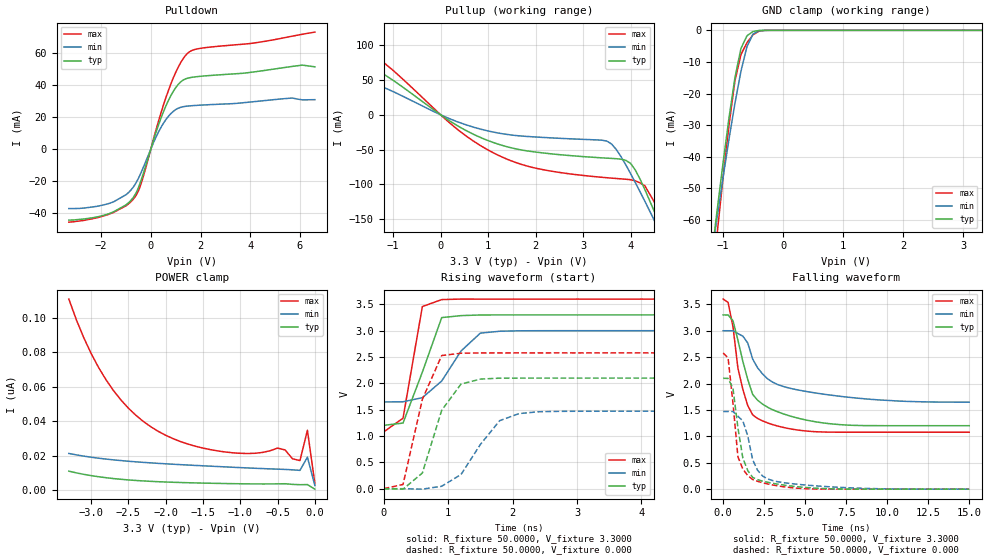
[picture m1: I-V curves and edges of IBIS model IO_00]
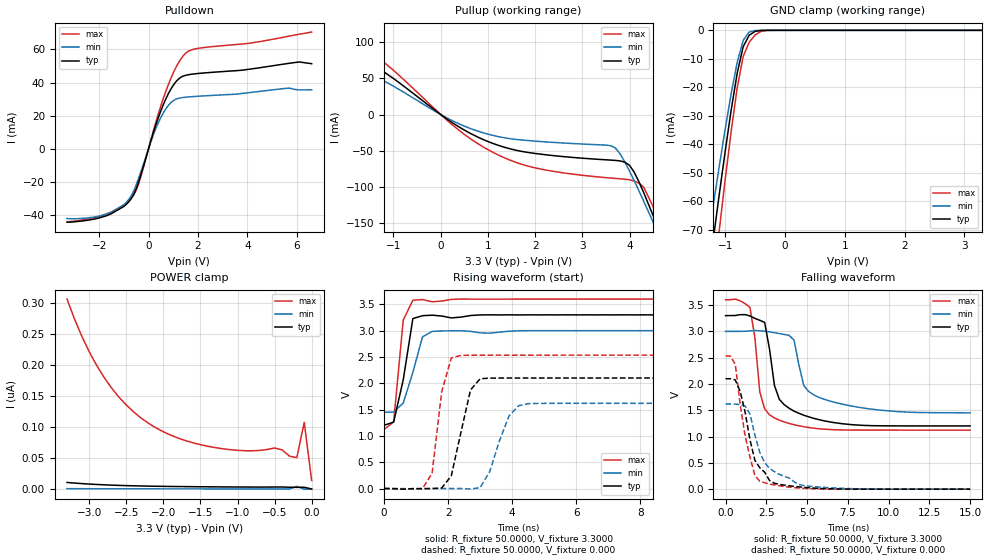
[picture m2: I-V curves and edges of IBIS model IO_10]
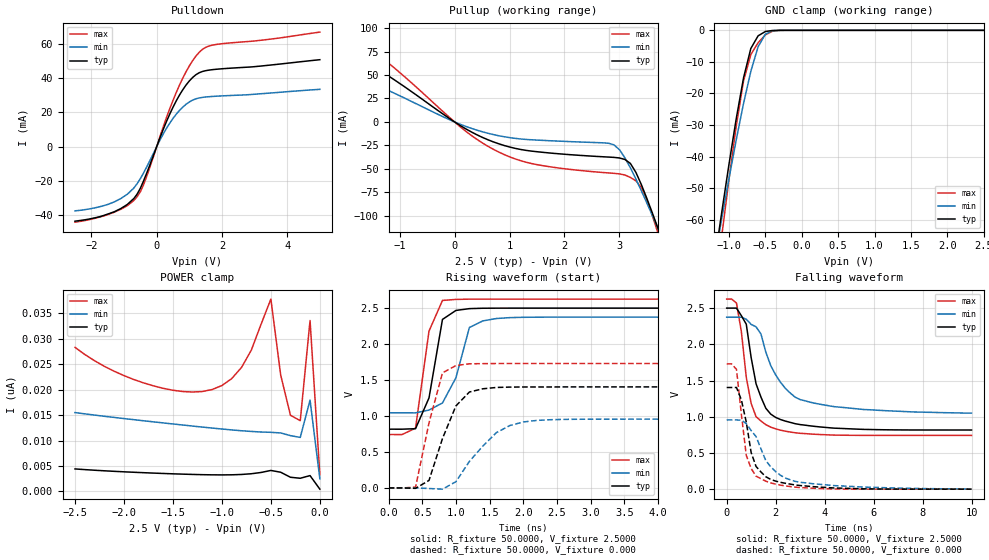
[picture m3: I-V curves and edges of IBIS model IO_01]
| Xilinx XC9500XV IBIS File
[IBIS ver]   2.1
[File name]   xc9500xv.ibs
[File Rev]   0.2
[Date]   Mar. 6, 2001
[Source]   Hspice simulations
[Notes]   Xilinx IBIS model for XC9500XV I/O
|   The package models are provided for CS48, PC44, VQ44
|   TQ100, TQ144, CS144, PQ208, FG256, and CS280 package
|   types, with CS48 being selected as a default. Please
|   make your own selection of the packages by commenting
|   out the unused ones.
|   Control flag setting:
|   SLW=0 - fast slew rate
|   SLW=1 - slow slew rate
|   VIO=2 - 1.8V Vddio
|   VIO=1 - 2.5V Vddio
|   VIO=0 - 3.3V Vddio
|   COMMENTS: Models include process corners for MIN and MAX.
[Disclaimer]   The data in this model is derived from SPICE simulations
|   using modeling information extracted from the target pro-
|   cess. While a great deal of care has been take to provide
|   information that is accurate, this model is considered
|   preliminary as it has not been verified by actual silicon
|   measurement. Treat the data in this model as preliminary
|   until actual silicon verification is performed.
[Copyright]   Copyright 2001, Xilinx Inc., All rights reserved
|   Component XC9500XV
|   >>> Make Your Selection of the Package type Below <<<
[Component]   XC9500XV
[Manufacturer]   Xilinx Inc.
[Package]
| For package type CS48:
| variable   typ   min   max
R_pkg   112.000m   98.0000m   126.000m
L_pkg   2.1000nH   1.8000nH   2.4000nH
C_pkg   0.2500pF   0.2000pF   0.3000pF
| For package type PC44:
| variable   typ   min   max
|R_pkg   67.5000m   66.0000m   69.0000m
|L_pkg   3.9500nH   3.6000nH   4.3000nH
|C_pkg   0.9000pF   0.8000pF   1.0000pF
| For package type VQ44:
| variable   typ   min   max
|R_pkg   57.0000m   54.0000m   60.0000m
|L_pkg   2.2500nH   2.1000nH   2.4000nH
|C_pkg   0.3000pF   0.3000pF   0.3000pF
| For package type TQ100:
| variable   typ   min   max
|R_pkg   103.000m   98.0000m   108.000m
|L_pkg   5.3000nH   4.7000nH   5.9000nH
|C_pkg   0.5500pF   0.4000pF   0.7000pF
| For package type TQ144:
| variable   typ   min   max
|R_pkg   127.000m   117.000m   137.000m
|L_pkg   8.1500nH   7.1000nH   9.2000nH
|C_pkg   1.0500pF   0.8000pF   1.3000pF
| For package type CS144:
| variable   typ   min   max
|R_pkg   109.500m   76.0000m   143.000m
|L_pkg   2.2500nH   1.5000nH   3.0000nH
|C_pkg   0.2500pF   0.2000pF   0.3000pF
| For package type PQ208:
| variable   typ   min   max
|R_pkg   195.500m   195.000m   196.000m
|L_pkg   14.200nH   12.500nH   15.900nH
|C_pkg   1.8000pF   1.6000pF   2.0000pF
| For package type FG256:
| variable   typ   min   max
|R_pkg   185.500m   141.000m   230.000m
|L_pkg   4.8500nH   3.3000nH   6.4000nH
|C_pkg   0.7500pF   0.5000pF   1.0000pF
| For package type CS280:
| variable   typ   min   max
|R_pkg   259.500m   148.000m   371.000m
|L_pkg   5.8000nH   2.7000nH   8.9000nH
|C_pkg   0.5000pF   0.2000pF   0.8000pF
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[Pin]  signal_name   model_name   R_pin   L_pin   C_pin
io_0   io_0   IO_00   NA   NA   NA
io_1   io_1   IO_01   NA   NA   NA
io_2   io_2   IO_10   NA   NA   NA
io_3   io_3   IO_11   NA   NA   NA
io_4   io_4   IO_02   NA   NA   NA
io_5   io_5   IO_12   NA   NA   NA
VCCO   VCCO   POWER   NA   NA   NA
PGND   GND   GND   NA   NA   NA
| Models and submodels in the file (6): IO_00 (I/O), IO_10 (I/O), IO_01 (I/O), IO_11 (I/O), IO_02 (I/O), IO_12 (I/O)
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|   Model IO_00
[Model]   IO_00
Model_type   I/O
Polarity   Non-Inverting
Enable   Active-High
Vinl =   0.8000V
Vinh =   2.0000V
Vmeas =   1.5000V
Cref =  50.0000pF
Rref =   1.0000M
Vref =  0.000V
C_comp   1.8820pF   1.2910pF   2.4730pF
[Temperature Range]   25.0000   100.0000   0.000
[Voltage Range]   3.3000V   3.0000V   3.6000V
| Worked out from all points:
|   slope of the pulldown table from 0 to 0.495 V, typ, clamps not added: 21.7 ohm
|   slope of the pullup table from 0 to 0.495 V, typ, clamps not added: 23.3 ohm
|   GND clamp passes 1 mA (typ) near -0.55 V on its own axis
|   rising waveform, R_fixture 50.0000, V_fixture 3.3000: 20-80 % time 377ps typ, 522ps min, 214ps max; typ from 1.2 V to 3.3 V
|   rising waveform, R_fixture 50.0000, V_fixture 0.000: 20-80 % time 385ps typ, 511ps min, 351ps max; typ from 0 V to 2.1 V
|   falling waveform, R_fixture 50.0000, V_fixture 3.3000: 20-80 % time 1.51ns typ, 2.44ns min, 914ps max; typ from 3.3 V to 1.2 V
|   falling waveform, R_fixture 50.0000, V_fixture 0.000: 20-80 % time 721ps typ, 953ps min, 579ps max; typ from 2.1 V to 0 V
[Pulldown]
| voltage   I(typ)   I(min)   I(max)
-3.3V     -44.4mA    -37.2mA    -45.7mA
-1.5V     -39.2mA    -33mA      -39.6mA
-900mV    -33.61mA   -27.22mA   -34.3mA
-600mV    -27.65mA   -21.23mA   -29.11mA
-400mV    -19.86mA   -14.99mA   -22.06mA
200mV     10.04mA    7.201mA    11.53mA
600mV     26.71mA    18.26mA    31.83mA
1.1V      40.32mA    25.49mA    51.09mA
1.5V      44.33mA    26.86mA    60.13mA
2V        45.44mA    27.42mA    62.92mA
6.1V      52.41mA    30.72mA    71.7mA
6.6V      51.35mA    30.83mA    73.05mA
[Pullup]
| voltage   I(typ)   I(min)   I(max)
-3.3V     27.71mA    12.26mA    53.81mA
-2.5V     82.24mA    44.55mA    121.5mA
-2.3V     93.8mA     55.81mA    126.3mA
-1.7V     79.94mA    53.81mA    102.7mA
300mV     -13.55mA   -8.683mA   -18.05mA
1.2V      -42.02mA   -26.09mA   -57.83mA
3.5V      -62.42mA   -37.86mA   -90.63mA
4V        -69.96mA   -84.71mA   -93.48mA
4.3V      -107.6mA   -124.5mA   -102.2mA
4.5V      -139.2mA   -152.1mA   -125.6mA
4.7V      -172.1mA   -180mA     -161.3mA
6.6V      -491mA     -449mA     -534.4mA
[GND_clamp]
| voltage   I(typ)   I(min)   I(max)
-3.3V     -420.2mA   -364.8mA   -490.5mA
-1.2V     -73.41mA   -72.76mA   -83.75mA
-1.1V     -57.66mA   -59.66mA   -65.15mA
-1V       -42.38mA   -46.89mA   -47.13mA
-900mV    -27.9mA    -34.62mA   -30.25mA
-800mV    -15.03mA   -23.13mA   -16mA
-700mV    -5.736mA   -12.97mA   -7.676mA
-600mV    -1.742mA   -5.18mA    -3.915mA
-500mV    -371uA     -1.195mA   -1.433mA
-400mV    -43.14uA   -156.3uA   -255.7uA
-300mV    -2.671uA   -9.839uA   -22.16uA
3.3V      462pA      11.68nA    3.111nA
[POWER_clamp]
| voltage   I(typ)   I(min)   I(max)
-3.3V     10.92nA    21.19nA    110.8nA
-3.1V     9.067nA    19.64nA    88.41nA
-2.8V     7.101nA    17.92nA    63.87nA
-2.6V     6.191nA    17.05nA    52.17nA
-2.3V     5.238nA    16.01nA    39.75nA
-2V       4.618nA    15.18nA    31.72nA
-1.6V     4.086nA    14.24nA    25.36nA
-900mV    3.547nA    12.78nA    21.16nA
-500mV    3.553nA    12.08nA    24.31nA
-200mV    3.052nA    11.37nA    17.04nA
-100mV    3.12nA     19.04nA    34.64nA
0V        462pA      2.582nA    3.744nA
[Ramp]
| variable   typ   min   max
dV/dt_r   1.2600/0.3171n   0.8826/0.5251n   1.5468/0.2348n
dV/dt_f   1.2588/1.4787n   0.8112/2.5016n   1.5132/0.8154n
R_load = 50.0000
[Rising Waveform]
R_fixture = 50.0000
V_fixture = 3.3000
V_fixture_min = 3.0000
V_fixture_max = 3.6000
L_fixture = 0.000H
C_fixture = 0.000F
| time   V(typ)   V(min)   V(max)
0s        1.202V     1.647V     1.078V
300ps     1.246V     1.65V      1.338V
600ps     2.213V     1.728V     3.458V
900ps     3.248V     2.044V     3.59V
1.2ns     3.286V     2.614V     3.6V
1.5ns     3.298V     2.954V     3.599V
1.8ns     3.299V     2.989V     3.599V
2.7ns     3.3V       2.999V     3.599V
15ns      3.299V     3V         3.599V
[Rising Waveform]
R_fixture = 50.0000
V_fixture = 0.000
V_fixture_min = 0.000
V_fixture_max = 0.000
L_fixture = 0.000H
C_fixture = 0.000F
| time   V(typ)   V(min)   V(max)
0s        7.285uV    -1.674uV   37.74uV
300ps     -9.219mV   -254.7uV   79.99mV
600ps     297.3mV    -9.006mV   1.696V
900ps     1.488V     46.1mV     2.528V
1.2ns     1.986V     269.2mV    2.572V
1.5ns     2.081V     838.4mV    2.577V
1.8ns     2.099V     1.292V     2.577V
2.1ns     2.099V     1.425V     2.578V
2.4ns     2.099V     1.46V      2.577V
15ns      2.1V       1.471V     2.578V
[Falling Waveform]
R_fixture = 50.0000
V_fixture = 3.3000
V_fixture_min = 3.0000
V_fixture_max = 3.6000
L_fixture = 0.000H
C_fixture = 0.000F
| time   V(typ)   V(min)   V(max)
0s        3.3V       3V         3.6V
300ps     3.298V     3V         3.536V
600ps     3.189V     2.999V     3.072V
900ps     2.821V     2.946V     2.292V
1.2ns     2.421V     2.898V     1.889V
1.8ns     1.794V     2.462V     1.407V
2.1ns     1.684V     2.299V     1.338V
3ns       1.506V     2.029V     1.224V
5.1ns     1.306V     1.848V     1.1V
15ns      1.202V     1.648V     1.078V
[Falling Waveform]
R_fixture = 50.0000
V_fixture = 0.000
V_fixture_min = 0.000
V_fixture_max = 0.000
L_fixture = 0.000H
C_fixture = 0.000F
| time   V(typ)   V(min)   V(max)
0s        2.1V       1.471V     2.578V
300ps     2.097V     1.471V     2.486V
600ps     1.907V     1.47V      1.623V
900ps     1.162V     1.381V     612.7mV
1.2ns     586.1mV    1.293V     381mV
1.5ns     351.2mV    1.008V     255.1mV
1.8ns     222.8mV    553.8mV    183mV
2.4ns     152.3mV    250.2mV    122.1mV
3.9ns     69.47mV    114.2mV    37.16mV
15ns      -2.014uV   295.5uV    8.128uV
|   Model IO_10
[Model]   IO_10
Model_type   I/O
Polarity   Non-Inverting
Enable   Active-High
Vinl =   0.8000V
Vinh =   2.0000V
Vmeas =   1.6500V
Cref =  50.0000pF
Rref =   1.0000M
Vref =  0.000V
C_comp   1.8820pF   1.2910pF   2.4730pF
[Temperature Range]   25.0000   100.0000   0.000
[Voltage Range]   3.3000V   3.0000V   3.6000V
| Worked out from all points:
|   slope of the pulldown table from 0 to 0.495 V, typ, clamps not added: 21.7 ohm
|   slope of the pullup table from 0 to 0.495 V, typ, clamps not added: 23.3 ohm
|   GND clamp passes 1 mA (typ) near -0.55 V on its own axis
|   rising waveform, R_fixture 50.0000, V_fixture 3.3000: 20-80 % time 376ps typ, 446ps min, 230ps max; typ from 1.2 V to 3.3 V
|   rising waveform, R_fixture 50.0000, V_fixture 0.000: 20-80 % time 463ps typ, 548ps min, 346ps max; typ from 0 V to 2.1 V
|   falling waveform, R_fixture 50.0000, V_fixture 3.3000: 20-80 % time 984ps typ, 1.33ns min, 632ps max; typ from 3.3 V to 1.2 V
|   falling waveform, R_fixture 50.0000, V_fixture 0.000: 20-80 % time 1.04ns typ, 1.44ns min, 854ps max; typ from 2.1 V to 0 V
[Pulldown]
| voltage   I(typ)   I(min)   I(max)
-3.3V     -44.4mA    -42.2mA    -44.2mA
-1.5V     -39.2mA    -38.4mA    -38.2mA
-900mV    -33.61mA   -32.45mA   -32.86mA
-600mV    -27.65mA   -25.55mA   -27.81mA
-300mV    -15.14mA   -13.43mA   -16.31mA
200mV     10.04mA    8.602mA    11.05mA
600mV     26.71mA    21.75mA    30.48mA
1.1V      40.32mA    29.88mA    48.89mA
1.5V      44.33mA    31.12mA    57.69mA
2V        45.44mA    31.7mA     60.62mA
5.7V      51.62mA    36.6mA     68.05mA
6.6V      51.35mA    35.6mA     70.46mA
[Pullup]
| voltage   I(typ)   I(min)   I(max)
-3.3V     27.71mA    12.83mA    54.63mA
-2.9V     53.58mA    22.01mA    86.38mA
-2.5V     82.24mA    49.56mA    116.8mA
-2.1V     92.52mA    70.56mA    114.9mA
400mV     -17.59mA   -13.18mA   -22.36mA
1.2V      -42.02mA   -30.17mA   -55.15mA
3.7V      -63.23mA   -46.15mA   -88.06mA
4V        -69.96mA   -77.93mA   -89.91mA
4.3V      -107.6mA   -119.4mA   -100.1mA
4.5V      -139.2mA   -148.2mA   -127mA
4.7V      -172.1mA   -177.4mA   -162.7mA
6.6V      -491mA     -457.1mA   -531.8mA
[GND_clamp]
| voltage   I(typ)   I(min)   I(max)
-3.3V     -420.2mA   -365.6mA   -490.8mA
-1.3V     -89.45mA   -75.32mA   -107.4mA
-1.2V     -73.41mA   -61.39mA   -88.65mA
-1.1V     -57.66mA   -47.75mA   -70.24mA
-1V       -42.38mA   -34.57mA   -52.33mA
-900mV    -27.9mA    -22.16mA   -35.32mA
-800mV    -15.03mA   -11.25mA   -20.15mA
-700mV    -5.736mA   -3.528mA   -9.193mA
-600mV    -1.742mA   -608.5uA   -4.204mA
-500mV    -371uA     -59.88uA   -1.634mA
-300mV    -2.671uA   -152.1nA   -37.23uA
3.3V      461.9pA    422.7pA    11.33nA
[POWER_clamp]
| voltage   I(typ)   I(min)   I(max)
-3.3V     10.91nA    933.2pA    305.8nA
-3.1V     9.067nA    856.3pA    245.9nA
-2.8V     7.101nA    768.9pA    179.9nA
-2.6V     6.191nA    724.5pA    148.2nA
-2.3V     5.238nA    670.2pA    114.4nA
-2V       4.618nA    625.6pA    92.38nA
-1.6V     4.086nA    573.1pA    74.67nA
-1V       3.6nA      500.6pA    62.56nA
-500mV    3.553nA    444.3pA    66.33nA
-200mV    3.052nA    4.621nA    50.74nA
-100mV    3.12nA     143.7pA    107.6nA
0V        461.8pA    109.6pA    14.14nA
[Ramp]
| variable   typ   min   max
dV/dt_r   1.2600/0.4174n   0.9714/0.5334n   1.5204/0.3030n
dV/dt_f   1.2588/0.9506n   0.9294/1.2765n   1.4868/0.5669n
R_load = 50.0000
[Rising Waveform]
R_fixture = 50.0000
V_fixture = 3.3000
V_fixture_min = 3.0000
V_fixture_max = 3.6000
L_fixture = 0.000H
C_fixture = 0.000F
| time   V(typ)   V(min)   V(max)
0s        1.202V     1.448V     1.122V
300ps     1.262V     1.453V     1.267V
600ps     2.067V     1.625V     3.203V
900ps     3.228V     2.207V     3.577V
1.2ns     3.284V     2.881V     3.591V
1.5ns     3.294V     2.984V     3.548V
2.1ns     3.242V     2.997V     3.594V
3.3ns     3.3V       2.951V     3.599V
4.5ns     3.3V       2.999V     3.599V
15ns      3.3V       3V         3.6V
[Rising Waveform]
R_fixture = 50.0000
V_fixture = 0.000
V_fixture_min = 0.000
V_fixture_max = 0.000
L_fixture = 0.000H
C_fixture = 0.000F
| time   V(typ)   V(min)   V(max)
0s        8.335uV    -3.113uV   50.68uV
1.2ns     -1.694mV   -3.592mV   -2.629mV
1.5ns     -582.1uV   -325.1uV   290.8mV
1.8ns     9.154mV    -54.68uV   1.839V
2.1ns     241.8mV    -10.28uV   2.482V
2.7ns     1.873V     -9.161mV   2.533V
3ns       2.086V     15.78mV    2.534V
3.9ns     2.099V     1.377V     2.534V
4.2ns     2.099V     1.573V     2.534V
15ns      2.1V       1.619V     2.534V
[Falling Waveform]
R_fixture = 50.0000
V_fixture = 3.3000
V_fixture_min = 3.0000
V_fixture_max = 3.6000
L_fixture = 0.000H
C_fixture = 0.000F
| time   V(typ)   V(min)   V(max)
0s        3.3V       3V         3.6V
1.5ns     3.294V     3.01V      3.455V
1.8ns     3.248V     3.017V     2.883V
2.1ns     3.211V     3.011V     1.851V
2.4ns     3.171V     3.004V     1.527V
3ns       1.972V     2.975V     1.354V
4.2ns     1.484V     2.834V     1.226V
4.8ns     1.405V     1.97V      1.187V
5.7ns     1.324V     1.748V     1.149V
15ns      1.202V     1.451V     1.122V
[Falling Waveform]
R_fixture = 50.0000
V_fixture = 0.000
V_fixture_min = 0.000
V_fixture_max = 0.000
L_fixture = 0.000H
C_fixture = 0.000F
| time   V(typ)   V(min)   V(max)
0s        2.1V       1.619V     2.534V
600ps     2.076V     1.618V     2.372V
900ps     1.859V     1.607V     1.613V
1.2ns     1.467V     1.581V     1.017V
1.5ns     938.8mV    1.429V     613.1mV
1.8ns     549.6mV    1.028V     259.7mV
2.1ns     407.3mV    701.2mV    152.1mV
3ns       111mV      330.4mV    81.19mV
4.8ns     34.49mV    68.61mV    15.63mV
15ns      -21.18uV   190.5uV    -17.78uV
|   Model IO_01
[Model]   IO_01
Model_type   I/O
Polarity   Non-Inverting
Enable   Active-High
Vinl =   0.8000V
Vinh =   2.0000V
Vmeas =   1.6500V
Cref =  50.0000pF
Rref =   1.0000M
Vref =  0.000V
C_comp   1.8820pF   1.2910pF   2.4730pF
[Temperature Range]   25.0000   100.0000   0.000
[Voltage Range]   2.5000V   2.3750V   2.6250V
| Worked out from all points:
|   slope of the pulldown table from 0 to 0.375 V, typ, clamps not added: 21 ohm
|   slope of the pullup table from 0 to 0.375 V, typ, clamps not added: 29.3 ohm
|   GND clamp passes 1 mA (typ) near -0.55 V on its own axis
|   rising waveform, R_fixture 50.0000, V_fixture 2.5000: 20-80 % time 213ps typ, 291ps min, 190ps max; typ from 0.817 V to 2.5 V
|   rising waveform, R_fixture 50.0000, V_fixture 0.000: 20-80 % time 332ps typ, 522ps min, 263ps max; typ from 0 V to 1.4 V
|   falling waveform, R_fixture 50.0000, V_fixture 2.5000: 20-80 % time 703ps typ, 1.21ns min, 507ps max; typ from 2.5 V to 0.817 V
|   falling waveform, R_fixture 50.0000, V_fixture 0.000: 20-80 % time 613ps typ, 1.09ns min, 445ps max; typ from 1.4 V to 0 V
[Pulldown]
| voltage   I(typ)   I(min)   I(max)
-2.5V     -43.3mA    -37.3mA    -43.9mA
-1.9V     -41.4mA    -35.6mA    -41.7mA
-1.3V     -37.85mA   -32.1mA    -38.1mA
-900mV    -33.61mA   -27.65mA   -34.3mA
-600mV    -27.65mA   -21.57mA   -29.14mA
-400mV    -19.86mA   -15.23mA   -22.08mA
200mV     10.04mA    7.385mA    11.51mA
600mV     26.71mA    18.98mA    31.58mA
1V        38.31mA    26.1mA     47.05mA
1.4V      43.85mA    28.77mA    56.7mA
1.8V      45.11mA    29.44mA    59.52mA
5V        50.73mA    33.47mA    66.81mA
[Pullup]
| voltage   I(typ)   I(min)   I(max)
-2.5V     70.1mA     45.22mA    94.12mA
-2.3V     77.89mA    51.6mA     101.4mA
-1.7V     66.38mA    45.58mA    84.64mA
200mV     -7.268mA   -4.674mA   -9.775mA
800mV     -23.24mA   -14.68mA   -32.02mA
1.5V      -31.78mA   -19.37mA   -45.55mA
2.9V      -37.82mA   -24.44mA   -54.84mA
3V        -38.44mA   -29.63mA   -55.39mA
3.2V      -44.33mA   -49.07mA   -59.2mA
3.4V      -67.03mA   -73.55mA   -69.94mA
3.7V      -113.3mA   -113.4mA   -118.3mA
5V        -330.3mA   -295.9mA   -372.6mA
[GND_clamp]
| voltage   I(typ)   I(min)   I(max)
-2.5V     -287.9mA   -252.7mA   -335.8mA
-1.2V     -73.41mA   -72.77mA   -83.79mA
-1.1V     -57.66mA   -59.67mA   -65.18mA
-1V       -42.38mA   -46.9mA    -47.16mA
-900mV    -27.9mA    -34.63mA   -30.27mA
-800mV    -15.03mA   -23.14mA   -16.01mA
-700mV    -5.735mA   -12.98mA   -7.684mA
-600mV    -1.742mA   -5.184mA   -3.919mA
-500mV    -371uA     -1.196mA   -1.434mA
-400mV    -43.13uA   -156.3uA   -255.7uA
-300mV    -2.669uA   -9.838uA   -22.12uA
2.5V      433pA      34.5nA     2.849nA
[POWER_clamp]
| voltage   I(typ)   I(min)   I(max)
-2.5V     4.412nA    15.49nA    28.31nA
-1.8V     3.673nA    13.88nA    21.33nA
-1.4V     3.387nA    13.05nA    19.63nA
-1.1V     3.251nA    12.45nA    20.02nA
-800mV    3.323nA    11.92nA    24.36nA
-700mV    3.464nA    11.78nA    27.76nA
-500mV    4.114nA    11.61nA    37.81nA
-400mV    3.762nA    11.49nA    22.88nA
-300mV    2.774nA    10.96nA    14.96nA
-200mV    2.578nA    10.61nA    13.9nA
-100mV    3.101nA    17.95nA    33.59nA
0V        433.1pA    2.482nA    3.286nA
[Ramp]
| variable   typ   min   max
dV/dt_r   0.8424/0.2731n   0.5735/0.4376n   1.0380/0.1864n
dV/dt_f   1.0099/0.6346n   0.7950/1.2162n   1.1296/0.4590n
R_load = 50.0000
[Rising Waveform]
R_fixture = 50.0000
V_fixture = 2.5000
V_fixture_min = 2.3750
V_fixture_max = 2.6250
L_fixture = 0.000H
C_fixture = 0.000F
| time   V(typ)   V(min)   V(max)
0s        816.6mV    1.044V     742.2mV
200ps     816.5mV    1.044V     741.9mV
400ps     823.5mV    1.044V     830.6mV
600ps     1.251V     1.082V     2.18V
800ps     2.342V     1.181V     2.606V
1ns       2.467V     1.532V     2.62V
1.2ns     2.492V     2.23V      2.624V
1.4ns     2.498V     2.321V     2.624V
1.6ns     2.498V     2.354V     2.624V
10ns      2.5V       2.374V     2.625V
[Rising Waveform]
R_fixture = 50.0000
V_fixture = 0.000
V_fixture_min = 0.000
V_fixture_max = 0.000
L_fixture = 0.000H
C_fixture = 0.000F
| time   V(typ)   V(min)   V(max)
0s        0V         0V         0V
400ps     -5.789mV   -115.9uV   10.9mV
600ps     104.4mV    -7.723mV   903.1mV
800ps     686.3mV    -17.15mV   1.599V
1ns       1.14V      86.7mV     1.701V
1.2ns     1.333V     368.9mV    1.725V
1.6ns     1.397V     768mV      1.729V
1.8ns     1.401V     867.2mV    1.729V
2.2ns     1.403V     938.5mV    1.729V
10ns      1.404V     955.8mV    1.73V
[Falling Waveform]
R_fixture = 50.0000
V_fixture = 2.5000
V_fixture_min = 2.3750
V_fixture_max = 2.6250
L_fixture = 0.000H
C_fixture = 0.000F
| time   V(typ)   V(min)   V(max)
0s        2.5V       2.375V     2.625V
400ps     2.5V       2.375V     2.571V
600ps     2.395V     2.374V     2.174V
800ps     2.278V     2.346V     1.545V
1ns       1.815V     2.275V     1.182V
1.2ns     1.455V     2.241V     1.001V
1.6ns     1.117V     1.891V     890mV
2.2ns     961.6mV    1.474V     814.4mV
3ns       891.8mV    1.237V     771.4mV
10ns      816.8mV    1.05V      742.3mV
[Falling Waveform]
R_fixture = 50.0000
V_fixture = 0.000
V_fixture_min = 0.000
V_fixture_max = 0.000
L_fixture = 0.000H
C_fixture = 0.000F
| time   V(typ)   V(min)   V(max)
0s        1.404V     955.8mV    1.73V
400ps     1.404V     955.8mV    1.654V
600ps     1.234V     952.8mV    1.035V
800ps     926mV      905mV      466.2mV
1ns       504.7mV    809.7mV    284.2mV
1.4ns     237.4mV    556.4mV    144.1mV
1.6ns     171.5mV    393.2mV    110mV
2ns       111.2mV    242.6mV    69.14mV
2.8ns     58mV       107.5mV    27.89mV
10ns      195.1uV    2.1mV      76.15uV
